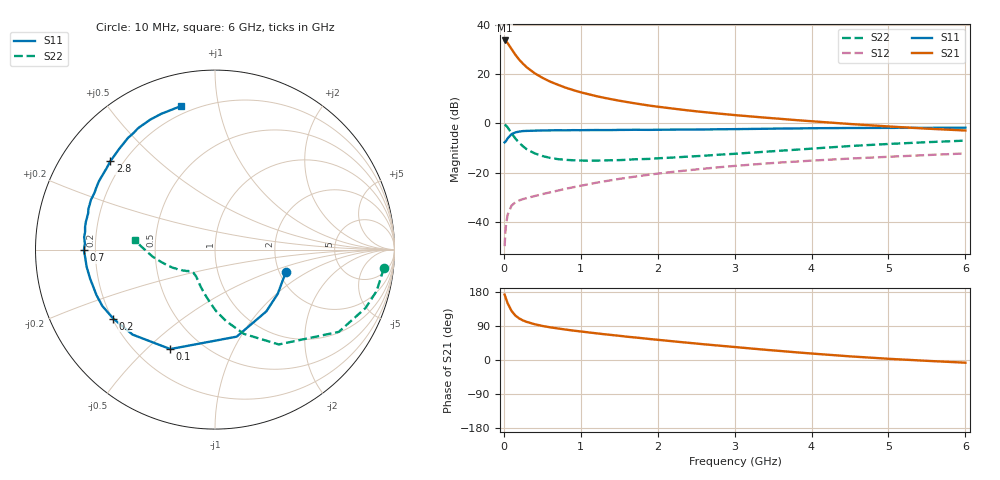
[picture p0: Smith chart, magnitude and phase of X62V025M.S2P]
! SIEMENS Small Signal Semiconductors
! BFP193W
! Si NPN RF Bipolar Junction Transistor in SOT343
! VCE = 2 V  IC = 25 mA
! Common Emitter S-Parameters:  April 1994
# GHz  S  MA  R  50
!  f  S11  S21  S12  S22
! GHz  MAG  ANG  MAG  ANG  MAG  ANG  MAG  ANG
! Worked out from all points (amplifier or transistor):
!   40 points, 10 MHz to 6 GHz, reference 50 ohm
!   highest |S21| = 33.6 dB at 10 MHz (marker M1)
!   |S21| within 3 dB of that: start of sweep to 90.1 MHz
!   unconditionally stable (mu >= 1): 795.4 MHz to 3.969 GHz
!   at 200 MHz: K = 0.42, MSG = 28.4 dB, |S12| = -31.1 dB
!   at 1.5 GHz: K = 1.12, MAG = 13.7 dB, |S12| = -22.4 dB
!   at 6 GHz: K = 0.93, MSG = 4.6 dB, |S12| = -12.1 dB
!   S11 on the Smith chart (normalised r, x): 10 MHz: 2.16, -0.66; 100 MHz: 0.34, -0.59; 200 MHz: 0.20, -0.29; 700 MHz: 0.16, -0.00; 2.8 GHz: 0.15, +0.36; 6 GHz: 0.16, +0.78
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0.01  0.414 -17.8  47.68 172.6  0.0033 83.9  0.9465 -6.3
0.02  0.4276 -35.1  46.98 166.8  0.0064 77.9  0.9295 -14.4
0.03  0.4476 -50.3  45.85 160.7  0.0094 75.1  0.8998 -21.2
0.05  0.4998 -76.0  41.99 149.4  0.0144 64.4  0.8281 -33.6
0.1  0.6076 -114.2  31.98 129.5  0.0218 50.2  0.6367 -56.1
0.15  0.6596 -134.1  24.5 117.2  0.0255 43.1  0.4962 -71.1
0.2  0.6849 -145.9  19.45 109.6  0.0278 40.7  0.4037 -81.1
0.25  0.702 -153.4  16.09 104.3  0.0296 39.6  0.3447 -88.7
0.3  0.7073 -159.0  13.58 100.4  0.031 40.6  0.2996 -94.9
0.4  0.7144 -166.9  10.38 94.4  0.034 41.8  0.2487 -104.3
0.5  0.7216 -172.4  8.401 89.9  0.0372 44.3  0.2201 -111.5
0.6  0.7247 -176.6  7.027 86.3  0.0404 46.6  0.2014 -117.1
0.7  0.7304 -179.8  6.084 83.3  0.0438 49.1  0.1902 -121.4
0.9  0.7324 174.5  4.739 77.7  0.0512 52.1  0.1802 -127.6
1.1  0.7348 170.1  3.905 72.8  0.0589 54.2  0.1767 -132.1
1.6  0.7419 160.2  2.714 61.5  0.0796 56.4  0.1841 -138.3
2.2  0.7504 149.7  1.996 49.3  0.105 55.4  0.2045 -145.2
2.8  0.7633 139.8  1.582 37.9  0.1302 52.5  0.234 -151.5
3.2  0.7744 133.6  1.391 30.6  0.1463 50.0  0.2559 -156.7
4.5  0.8092 116.5  0.975 9.6  0.1949 41.2  0.3494 -173.5
5.5  0.8153 107.8  0.785 -2.2  0.2294 34.8  0.418 176.8
6  0.8216 103.5  0.72 -7.1  0.2475 32.0  0.4495 173.0
